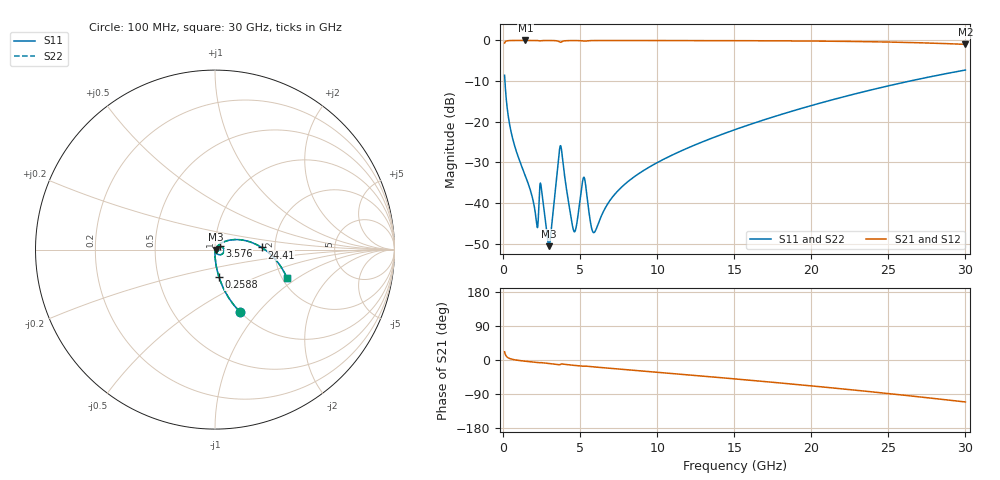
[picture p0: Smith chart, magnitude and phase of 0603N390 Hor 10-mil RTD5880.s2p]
# GHz S MA R 50
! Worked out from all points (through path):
!   3201 points, 100 MHz to 30 GHz, reference 50 ohm
!   highest |S21| = -0.01 dB at 1.446 GHz (marker M1); lowest = -1.0 dB at 30 GHz (marker M2)
!   group delay of S21, straight-line fit = 10.3 ps
!   lowest |S11| = -50.6 dB at 2.978 GHz (marker M3), VSWR 1.01, Z = 50.3 - j0.0658 ohm
!   |S11| at or under -10 dB: 120.6 MHz to 26.39 GHz (26.27 GHz wide, 198 % of centre)
!   |S22| runs from -50.6 to -7.3 dB; largest |S21 - S12| = 0
!   S11 on the Smith chart (normalised r, x): 100 MHz: 1.00, -0.80; 258.8 MHz: 1.00, -0.31; 3.576 GHz: 1.05, +0.04; 24.41 GHz: 1.70, +0.04; 30 GHz: 2.12, -0.83
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0.1  0.3731 -68.3  0.9274 21.6  0.9274 21.6  0.3731 -68.3
0.2588437  0.1527 -81.8  0.9878 8.0  0.9878 8.0  0.1527 -81.8
0.6512813  0.05911 -87.9  0.9975 1.4  0.9975 1.4  0.05911 -87.9
1.4455  0.02158 -90.2  0.9986 -3.2  0.9986 -3.2  0.02158 -90.2
2.155625  0.006077 -70.4  0.9973 -6.4  0.9973 -6.4  0.006077 -70.4
2.501344  0.0143 -63.1  0.9919 -7.1  0.9919 -7.1  0.0143 -63.1
2.977875  0.002946 -12.8  0.997 -9.2  0.997 -9.2  0.002946 -12.8
3.575875  0.03128 35.9  0.9789 -12.4  0.9789 -12.4  0.03128 35.9
3.800125  0.04389 -39.0  0.9611 -10.5  0.9611 -10.5  0.04389 -39.0
4.603688  0.004475 -24.5  0.9955 -14.2  0.9955 -14.2  0.004475 -24.5
4.781219  0.005547 13.9  0.9951 -14.9  0.9951 -14.9  0.005547 13.9
5.089563  0.01497 22.6  0.9882 -16.2  0.9882 -16.2  0.01497 22.6
5.304469  0.0193 -25.1  0.9808 -16.2  0.9808 -16.2  0.0193 -25.1
5.696906  0.005423 -32.2  0.9947 -17.5  0.9947 -17.5  0.005423 -32.2
5.921156  0.004348 4.7  0.9959 -18.3  0.9959 -18.3  0.004348 4.7
7.397469  0.01379 54.0  0.9968 -23.5  0.9968 -23.5  0.01379 54.0
10.06978  0.03189 51.7  0.9961 -32.6  0.9961 -32.6  0.03189 51.7
15.05  0.07994 37.2  0.9926 -49.9  0.9926 -49.9  0.07994 37.2
20.03956  0.1587 19.8  0.9821 -68.4  0.9821 -68.4  0.1587 19.8
24.41244  0.26 2.6  0.9593 -86.1  0.9593 -86.1  0.26 2.6
25.01978  0.2766 0.1  0.9546 -88.6  0.9546 -88.6  0.2766 0.1
30  0.4322 -21.7  0.8941 -110.8  0.8941 -110.8  0.4322 -21.7
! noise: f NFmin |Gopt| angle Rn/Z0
0.1  0.0002889  0.9175  0.3948  0.0007734
3.417  0.007593  0.8944  10.55  0.01554
6.743  0.006712  0.78  20.72  0.006053
10.06  0.008359  0.7447  30.64  0.006126
13.39  0.01033  0.7312  40.34  0.00677
16.7  0.01235  0.7253  49.72  0.007391
20.03  0.01446  0.7243  58.79  0.007969
23.35  0.0167  0.7271  67.48  0.008505
26.67  0.01912  0.7327  75.86  0.009008
30  0.02179  0.7408  83.9  0.009486
